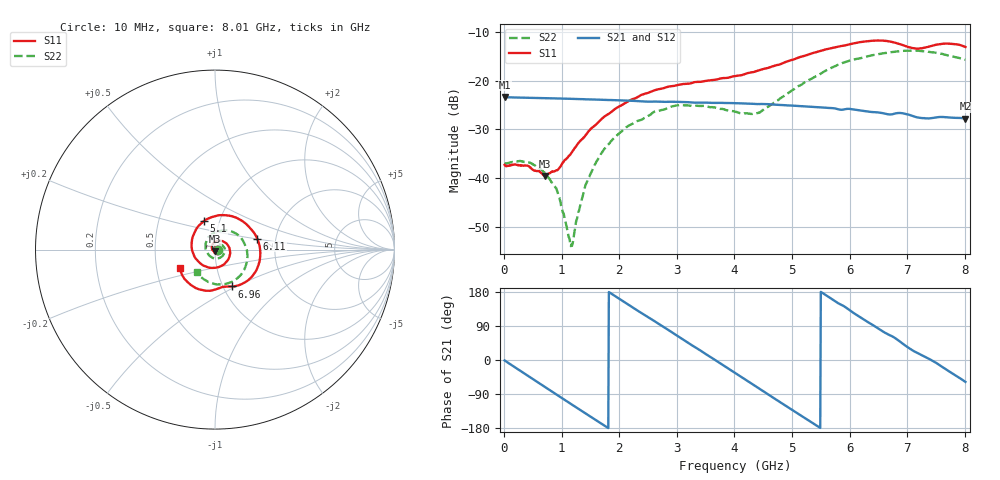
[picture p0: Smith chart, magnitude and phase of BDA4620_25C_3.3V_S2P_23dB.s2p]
!Agilent Technologies,E5071B,MY42404982,A.09.10
!Date: Wed May 06 08:53:47 2026
!Data & Calibration Information:
!Freq	S11:SOLT2(ON)	S21:SOLT2(ON)	S12:SOLT2(ON)	S22:SOLT2(ON)
# Hz S RI R 50
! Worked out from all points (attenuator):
!   801 points, 10 MHz to 8.01 GHz, reference 50 ohm
!   highest |S21| = -23.39 dB at 10 MHz (marker M1); lowest = -27.8 dB at 8.01 GHz (marker M2)
!   lowest |S11| = -39.5 dB at 710 MHz (marker M3), VSWR 1.02, Z = 49.8 - j1.04 ohm
!   |S11| at or under -10 dB: start of sweep to end of sweep
!   |S22| runs from -53.9 to -13.8 dB; largest |S21 - S12| = 0.00032
!   S11 on the Smith chart (normalised r, x): 10 MHz: 1.03, -0.00; 5.1 GHz: 0.84, +0.28; 6.11 GHz: 1.60, +0.21; 6.96 GHz: 1.10, -0.48; 8.01 GHz: 0.66, -0.15
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1e7  0.0136 -0.000839  0.0677 -0.00142  0.0677 -0.00144  0.0141 -0.000449
4.4e8  0.00858 -0.0099  0.0477 -0.0466  0.0477 -0.0466  0.0134 -0.00517
7.1e8  -0.00161 -0.0104  0.0213 -0.0626  0.0213 -0.0627  0.00862 -0.00723
9.3e8  -0.0106 -0.00574  -0.00346 -0.0655  -0.00355 -0.0656  0.00347 -0.00634
1.16e9  -0.0169 0.00551  -0.0283 -0.0585  -0.0284 -0.0585  -0.00163 -0.00117
1.2e9  -0.0175 0.00795  -0.0322 -0.0563  -0.0323 -0.0563  -0.00227 3.39e-05
1.35e9  -0.0177 0.0176  -0.0452 -0.0459  -0.0453 -0.0459  -0.0038 0.00463
1.53e9  -0.0131 0.0301  -0.0566 -0.0298  -0.0567 -0.0299  -0.00363 0.0114
1.77e9  0.00117 0.0437  -0.0631 -0.00462  -0.0632 -0.00471  0.000592 0.0207
2.15e9  0.0374 0.0483  -0.0522 0.034  -0.0522 0.0341  0.0171 0.0295
2.68e9  0.0812 0.00638  -0.00617 0.0605  -0.00611 0.0606  0.0448 0.0197
3.08e9  0.0762 -0.0509  0.033 0.0505  0.0332 0.0505  0.0555 -0.0075
4.01e9  -0.0727 -0.0838  0.0486 -0.0328  0.0486 -0.0329  -0.0108 -0.0469
4.42e9  -0.127 -0.00568  0.0157 -0.0553  0.0156 -0.0553  -0.0451 -0.0129
5.1e9  -0.06 0.1598  -0.0429 -0.0344  -0.043 -0.0344  -0.0187 0.0848
5.35e9  0.0141 0.1898  -0.0521 -0.0132  -0.052 -0.0132  0.023 0.1028
5.69e9  0.1294 0.1725  -0.0494 0.017  -0.0494 0.017  0.0897 0.1017
6.11e9  0.2355 0.061  -0.025 0.0435  -0.025 0.0435  0.1613 0.0403
6.68e9  0.1905 -0.1659  0.0178 0.0412  0.0179 0.0413  0.1709 -0.0911
6.96e9  0.0959 -0.2052  0.0355 0.0286  0.0356 0.0287  0.1331 -0.1518
7.59e9  -0.0756 -0.2249  0.0406 -0.012  0.0407 -0.0119  -0.0214 -0.1871
8.01e9  -0.1946 -0.1048  0.0217 -0.0343  0.0218 -0.0344  -0.1029 -0.1272
